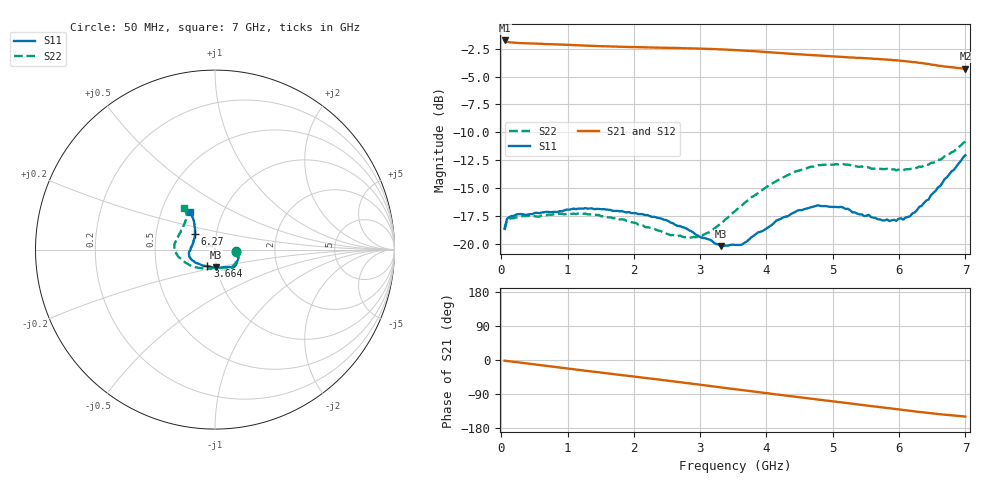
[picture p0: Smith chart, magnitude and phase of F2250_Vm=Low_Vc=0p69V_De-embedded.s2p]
! Integrated Device Technology
! Corporate Headquarters
! 6024 Silver Creek Valley Road
! San Jose, CA 95138  USA
! Phone:  1-408-284-8200
! Toll Free:  1-800-223-1366
! Webpage:  http://www.idt.com/
! Timing and RF Division
! 515 Groton Road, Suite 102
! Westford, MA 01886-6024
! Device:  F2250
! Description: Voltage Variable RF Attenuator
! Frequency:  50.0 -  6000.00 MHz
! Package:  3x3 mm Thin QFN Plastic Package: 16 pin
! Ports:  2 RF, 3 DC
!  Pin  1  = GND
!  Pin  2  = NC
!  Pin  3  = RF1  = Port 1
!  Pin  4  = NC
!  Pin  5  = GND
!  Pin  6  = GND
!  Pin  7  = GND
!  Pin  8  = GND
!  Pin  9  = NC
!  Pin 10  = RF2  = Port 2
!  Pin 11  = NC
!  Pin 12  = GND
!  Pin 13  = GND
!  Pin 14  = VCNTRL
!  Pin 15  = VDD
!  Pin 16  = VMODE
! Vcntrl:  0.690 Volts
! Vmode:  +0.000 Volts
! Vdd:  +3.30  Volts
! Current:  1.150 mA
! Data:  The device was measured on a the F2250 evaluation board which has
!  individual transmission lines to the RF pins.  Data was collected
!  using a calibrated network analyzer.  The evaluation board was
!  de-embedded using a TRL calibration technique.
!  The reference plane is the edge of the package pin.
! Misc:  SN 10
!  Action Tracker AT0258
! Date Measured:  2014-11-26
! Date:  2015-10-15  MJV
! Note:
!  Integrated Device Technology supplies this data as a sample of measured
!  data at the package pin for this product.  Your particular data for this
!  product may vary.
!  Data was taken at 25 degrees C.
!  Integrated Device Technology reserves the right to change this data at anytime.
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# GHz S dB R 50
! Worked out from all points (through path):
!   201 points, 50 MHz to 7 GHz, reference 50 ohm
!   highest |S21| = -1.77 dB at 50 MHz (marker M1); lowest = -4.3 dB at 7 GHz (marker M2)
!   group delay of S21, straight-line fit = 59.9 ps
!   lowest |S11| = -20.2 dB at 3.317 GHz (marker M3), VSWR 1.22, Z = 49.5 - j9.79 ohm
!   |S11| at or under -10 dB: start of sweep to end of sweep
!   |S22| runs from -19.4 to -10.8 dB; largest |S21 - S12| = 0.00089
!   S11 on the Smith chart (normalised r, x): 50 MHz: 1.27, -0.02; 3.664 GHz: 0.90, -0.17; 6.27 GHz: 0.79, +0.14; 7 GHz: 0.70, +0.31
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0.05  -18.57 -4.3  -1.77 -1.9  -1.77 -1.9  -18.73 -5.8
0.08475  -17.73 -4.6  -1.89 -2.5  -1.89 -2.5  -17.88 -5.6
0.2585  -17.29 -10.0  -2.00 -6.3  -2.00 -6.3  -17.58 -12.6
0.71025  -17.10 -23.9  -2.10 -16.2  -2.10 -16.2  -17.34 -29.9
1.2315  -16.81 -37.3  -2.23 -27.5  -2.22 -27.5  -17.28 -48.5
1.75275  -17.02 -44.1  -2.33 -38.4  -2.33 -38.4  -17.64 -59.9
2.37825  -17.66 -48.2  -2.42 -51.7  -2.42 -51.7  -18.79 -72.4
2.552  -18.05 -50.9  -2.43 -55.5  -2.43 -55.5  -19.19 -78.4
2.93425  -19.14 -62.5  -2.49 -63.9  -2.49 -63.9  -19.38 -97.9
3.14275  -19.58 -74.3  -2.54 -68.5  -2.53 -68.5  -18.91 -111.9
3.3165  -20.17 -87.1  -2.57 -72.4  -2.57 -72.4  -18.15 -122.6
3.525  -20.06 -103.3  -2.64 -77.0  -2.64 -77.1  -17.04 -134.4
3.664  -19.89 -114.8  -2.68 -80.2  -2.69 -80.2  -16.33 -141.0
4.1505  -17.88 -143.8  -2.87 -90.9  -2.87 -90.9  -14.34 -162.3
4.7065  -16.63 -162.9  -3.09 -102.9  -3.08 -102.9  -13.05 -177.6
5.1235  -16.65 -173.1  -3.23 -111.8  -3.23 -111.8  -12.86 172.9
5.471  -17.47 176.4  -3.35 -119.2  -3.35 -119.2  -13.14 165.3
5.85325  -17.92 162.1  -3.50 -127.3  -3.50 -127.3  -13.34 155.5
6.06175  -17.79 152.4  -3.61 -131.8  -3.61 -131.8  -13.40 149.3
6.27025  -16.94 141.7  -3.74 -136.3  -3.74 -136.3  -13.16 142.6
6.61775  -14.80 128.5  -4.04 -143.0  -4.04 -143.0  -12.44 131.0
7  -12.04 123.5  -4.31 -149.2  -4.30 -149.2  -10.81 126.5
